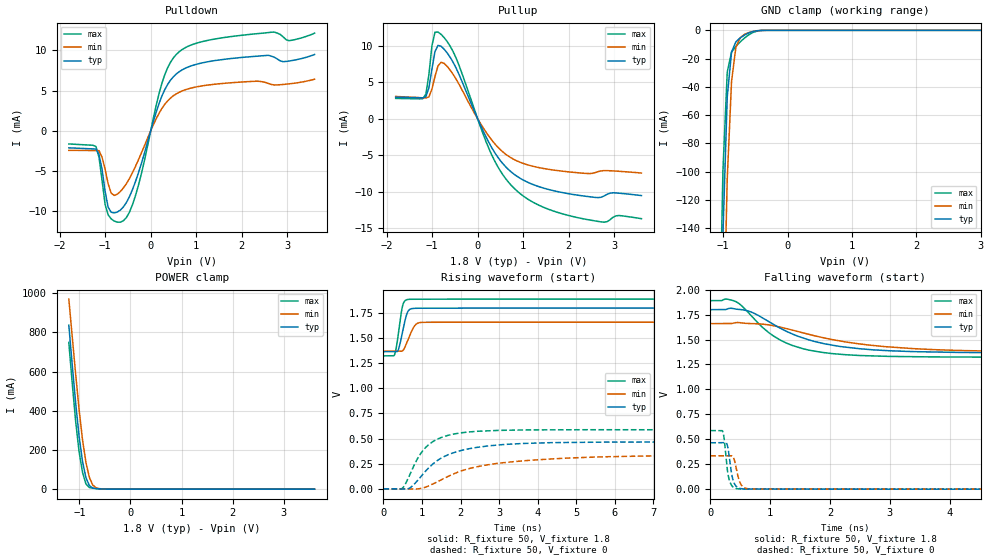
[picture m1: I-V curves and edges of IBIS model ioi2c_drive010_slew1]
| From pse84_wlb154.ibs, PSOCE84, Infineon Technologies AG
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[Model] ioi2c_drive010_slew1
Model_type I/O
Enable   Active-High
Vinl  =  0.54
Vinh  =  1.26
Vmeas =  0.9
Cref  =  15e-12
| Capacitance   typ   min   max
C_comp   8.55364e-13 8.30808e-13 8.84570e-13
| Variables   typ   min   max
[GND Clamp Reference]   0   0   0
[POWER Clamp Reference]   1.8   1.66   1.89
[Pulldown Reference]   0   0   0
[Pullup Reference]   1.8   1.66   1.89
[Temperature Range]   25   125   -40
[Voltage Range]   1.8   1.66   1.89
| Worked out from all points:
|   slope of the pulldown table from 0 to 0.27 V, typ, clamps not added: 58.4 ohm
|   slope of the pullup table from 0 to 0.27 V, typ, clamps not added: 76.8 ohm
|   GND clamp passes 1 mA (typ) near -0.55 V on its own axis
|   POWER clamp passes 1 mA (typ) near -0.55 V on its own axis
|   falling waveform, R_fixture 50, V_fixture 1.8: 20-80 % time 1.07ns typ, 1.58ns min, 763ps max; typ from 1.8 V to 1.37 V
|   falling waveform, R_fixture 50, V_fixture 0: 20-80 % time 73.1ps typ, 82.4ps min, 68.3ps max; typ from 0.465 V to 0 V
|   rising waveform, R_fixture 50, V_fixture 1.8: 20-80 % time 149ps typ, 196ps min, 126ps max; typ from 1.37 V to 1.8 V
|   rising waveform, R_fixture 50, V_fixture 0: 20-80 % time 1.02ns typ, 1.92ns min, 625ps max; typ from 0 V to 0.465 V
[GND Clamp]
| Voltage   I(typ)   I(min)   I(max)
-1.204V   -750.5mA   -844.3mA   -692.2mA
-1.07V    -311.8mA   -416.8mA   -250.3mA
-1.003V   -144.6mA   -236.7mA   -99.35mA
-936.6mV  -47.15mA   -105.3mA   -29.57mA
-869.7mV  -15.32mA   -36.11mA   -15.4mA
-802.8mV  -8.178mA   -12.13mA   -11.32mA
-735.9mV  -5.345mA   -5.294mA   -8.218mA
-669mV    -3.361mA   -2.852mA   -5.471mA
-535.2mV  -838.5uA   -772.4uA   -1.486mA
-401.4mV  -47.36uA   -84.85uA   -76.78uA
3.6V      0A         0A         0A
[POWER Clamp]
| Voltage   I(typ)   I(min)   I(max)
-1.204V   837.3mA    970.7mA    749.2mA
-1.137V   634.9mA    778.2mA    540.5mA
-1.07V    440.1mA    587.4mA    346.5mA
-1.003V   270mA      407mA      190.9mA
-936.6mV  141.8mA    252.7mA    85.92mA
-869.7mV  58.74mA    136.5mA    26.66mA
-802.8mV  18.35mA    60.36mA    8.197mA
-735.9mV  5.885mA    21mA       4.755mA
-669mV    2.866mA    6.628mA    3.138mA
-334.5mV  12.31uA    45.7uA     5.857uA
3.6V      0A         0A         0A
[Pulldown]
| Voltage   I(typ)   I(min)   I(max)
-1.8V     -2.132mA   -2.444mA   -1.643mA
-1.204V   -2.279mA   -2.463mA   -1.96mA
-1.07V    -4.767mA   -3.283mA   -6.143mA
-1.003V   -7.525mA   -4.772mA   -9.15mA
-936.6mV  -9.492mA   -6.579mA   -10.45mA
-802.8mV  -10.22mA   -8.048mA   -11.23mA
-669mV    -9.874mA   -7.568mA   -11.37mA
-401.4mV  -7.319mA   -5.22mA    -9.208mA
248.3mV   4.356mA    2.795mA    5.95mA
558.6mV   7.043mA    4.577mA    9.465mA
1.552V    8.83mA     5.862mA    11.53mA
3.6V      9.476mA    6.404mA    12.13mA
[Pullup]
| Voltage   I(typ)   I(min)   I(max)
-1.8V     2.946mA    3.055mA    2.787mA
-1.137V   3.017mA    2.847mA    3.365mA
-1.07V    4.244mA    3.001mA    6.052mA
-1.003V   6.848mA    4.069mA    10.02mA
-936.6mV  9.232mA    5.804mA    11.89mA
-869.7mV  10.07mA    7.26mA     11.9mA
-735.9mV  9.553mA    7.601mA    11.14mA
-468.3mV  6.898mA    5.392mA    8.266mA
372.4mV   -4.617mA   -3.408mA   -5.769mA
869mV     -7.921mA   -5.806mA   -9.94mA
2.191V    -10.49mA   -7.414mA   -13.57mA
3.6V      -10.56mA   -7.462mA   -13.73mA
[Ramp]
dV/dt_r   0.279116/1.01604n  0.200591/1.92042n  0.352378/0.625182n
dV/dt_f   0.260514/1.0707n  0.172747/1.58291n  0.339364/0.762999n
R_load = 50
[Falling Waveform]
R_fixture = 50
V_fixture = 1.8
V_fixture_min = 1.66
V_fixture_max = 1.89
| Time   V(typ)   V(min)   V(max)
0s        1.8V       1.66V      1.89V
270.2ps   1.803V     1.66V      1.906V
436.5ps   1.805V     1.67V      1.878V
721.9ps   1.766V     1.66V      1.713V
1.045ns   1.655V     1.64V      1.54V
1.364ns   1.558V     1.596V     1.442V
1.648ns   1.496V     1.551V     1.394V
2.723ns   1.397V     1.44V      1.336V
4.516ns   1.369V     1.386V     1.324V
800ns     1.366V     1.372V     1.324V
[Falling Waveform]
R_fixture = 50
V_fixture = 0
V_fixture_min = 0
V_fixture_max = 0
| Time   V(typ)   V(min)   V(max)
0s        465.2mV    334.3mV    587.3mV
208.9ps   465.1mV    334.3mV    578.1mV
232.7ps   465mV      334.3mV    501mV
285.8ps   438.4mV    334.3mV    190.9mV
322.5ps   298.8mV    334.2mV    81.69mV
371.4ps   110.7mV    331mV      26.11mV
486.8ps   8.914mV    79.32mV    2.141mV
557ps     1.876mV    18.12mV    1.292mV
1.202ns   544.6uV    617.6uV    403.4uV
800ns     11.23nV    709.4nV    4.431nV
[Rising Waveform]
R_fixture = 50
V_fixture = 1.8
V_fixture_min = 1.66
V_fixture_max = 1.89
| Time   V(typ)   V(min)   V(max)
0s        1.366V     1.372V     1.324V
291.4ps   1.366V     1.372V     1.337V
336.7ps   1.365V     1.372V     1.412V
395.8ps   1.395V     1.372V     1.565V
482.3ps   1.536V     1.371V     1.796V
557.4ps   1.672V     1.411V     1.873V
665.6ps   1.782V     1.513V     1.888V
876.6ps   1.798V     1.647V     1.888V
1.563ns   1.799V     1.659V     1.89V
800ns     1.8V       1.66V      1.89V
[Rising Waveform]
R_fixture = 50
V_fixture = 0
V_fixture_min = 0
V_fixture_max = 0
| Time   V(typ)   V(min)   V(max)
0s        11.24nV    709.2nV    4.431nV
492.3ps   -2.787mV   -481.2uV   5.144mV
698.9ps   11.59mV    -2.081mV   152.4mV
954.8ps   113.4mV    2.246mV    344.6mV
1.371ns   273.7mV    64.33mV    489.1mV
1.933ns   373mV      165.7mV    552.5mV
2.886ns   433.4mV    249.3mV    580.9mV
4.748ns   461.3mV    305.5mV    588.4mV
7.884ns   466.3mV    331.1mV    587.9mV
50ns      465.2mV    334.3mV    587.3mV
